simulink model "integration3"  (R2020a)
settings: Solver=ode45  StartTime=0.0  StopTime=3  RelTol=1e-3  EnableMultiTasking=on

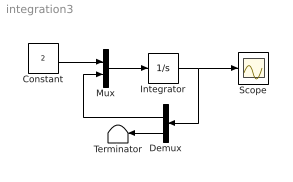
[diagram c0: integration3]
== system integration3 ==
  Constant : Constant  Value=2
  Demux : Demux  Outputs=[2,1]
  Integrator : Integrator  InitialCondition=[2,1,0]
  Mux : Mux  Inputs=2
  Scope : Scope
  Terminator : Terminator
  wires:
  Constant/1 -> Mux/1
  Mux/1 -> Integrator/1
  Integrator/1 -> Demux/1, Scope/1
  Demux/1 -> Mux/2
  Demux/2 -> Terminator/1
